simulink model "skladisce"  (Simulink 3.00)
settings: Solver=ode45  StartTime=0.0  StopTime=10.0  RelTol=1e-3
libraries: simulink3 x1

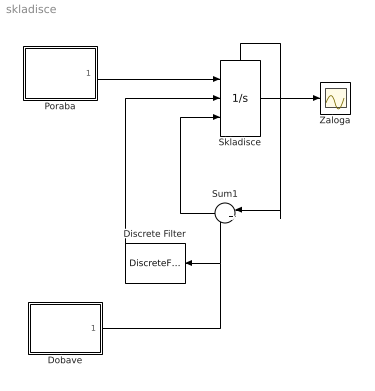
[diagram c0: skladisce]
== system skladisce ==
  Discrete Filter : DiscreteFilter  Orientation=left  Numerator=[1 -1]  Denominator=[1]  SampleTime=0.01
  Dobave : Subsystem
  Poraba : Subsystem
  Skladisce : Integrator  ExternalReset=rising  InitialConditionSource=external  InitialCondition=10  LimitOutput=off  UpperSaturationLimit=inf  LowerSaturationLimit=-inf  ShowSaturationPort=off  ShowStatePort=on  AbsoluteTolerance=auto
  Sum1 : Sum  Orientation=left  Inputs=|++  SaturateOnIntegerOverflow=on
  Zaloga : Scope
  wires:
  Skladisce/1 -> Zaloga/1
  Skladisce/State -> Sum1/1
  Sum1/1 -> Skladisce/3
  Poraba/1(Out1) -> Skladisce/1
  Dobave/1(Out1) -> Sum1/2, Discrete Filter/1
  Discrete Filter/1 -> Skladisce/2

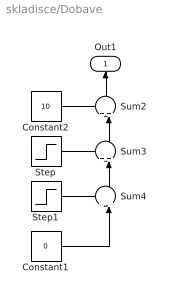
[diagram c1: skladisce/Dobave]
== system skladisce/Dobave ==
  Constant1 : Constant  Value=0
  Constant2 : Constant  Value=10
  Step : Step  Time=3  Before=0  After=3  SampleTime=0
  Step1 : Step  Time=7  Before=0  After=-3  SampleTime=0
  Sum2 : Sum  Orientation=up  Inputs=++|  SaturateOnIntegerOverflow=on
  Sum3 : Sum  Orientation=up  Inputs=++|  SaturateOnIntegerOverflow=on
  Sum4 : Sum  Orientation=up  Inputs=++|  SaturateOnIntegerOverflow=on
  Out1 : Outport  Orientation=up  Port=1
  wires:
  Constant2/1 -> Sum2/1
  Step/1 -> Sum3/1
  Sum3/1 -> Sum2/2
  Step1/1 -> Sum4/1
  Sum4/1 -> Sum3/2
  Constant1/1 -> Sum4/2
  Sum2/1 -> Out1/1

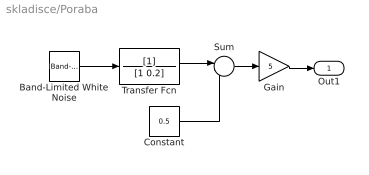
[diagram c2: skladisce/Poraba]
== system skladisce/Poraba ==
  Band-Limited White Noise : simulink3/Sources/Band-Limited White Noise  Cov=[0.1]  Ts=0.1  seed=[23341]
  Constant : Constant  Value=0.5
  Gain : Gain  Gain=5  SaturateOnIntegerOverflow=on
  Sum : Sum  Inputs=|--  SaturateOnIntegerOverflow=on
  Transfer Fcn : TransferFcn  Numerator=[1]  Denominator=[1 0.2]
  Out1 : Outport  Port=1
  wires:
  Transfer Fcn/1 -> Sum/1
  Sum/1 -> Gain/1
  Gain/1 -> Out1/1
  Constant/1 -> Sum/2
  Band-Limited White Noise/1 -> Transfer Fcn/1
